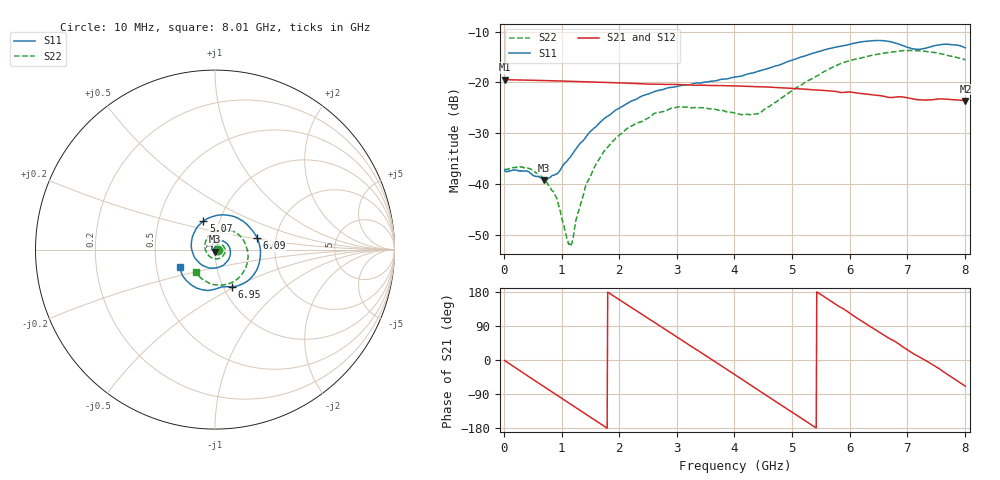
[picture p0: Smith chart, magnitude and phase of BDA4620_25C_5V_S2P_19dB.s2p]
!Agilent Technologies,E5071B,MY42404982,A.09.10
!Date: Wed May 06 09:02:22 2026
!Data & Calibration Information:
!Freq	S11:SOLT2(ON)	S21:SOLT2(ON)	S12:SOLT2(ON)	S22:SOLT2(ON)
# Hz S RI R 50
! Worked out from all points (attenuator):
!   801 points, 10 MHz to 8.01 GHz, reference 50 ohm
!   highest |S21| = -19.42 dB at 10 MHz (marker M1); lowest = -23.6 dB at 8.01 GHz (marker M2)
!   lowest |S11| = -39.2 dB at 700 MHz (marker M3), VSWR 1.02, Z = 49.8 - j1.08 ohm
!   |S11| at or under -10 dB: start of sweep to end of sweep
!   |S22| runs from -52.1 to -13.7 dB; largest |S21 - S12| = 0.00044
!   S11 on the Smith chart (normalised r, x): 10 MHz: 1.03, -0.00; 5.07 GHz: 0.84, +0.27; 6.09 GHz: 1.60, +0.22; 6.95 GHz: 1.10, -0.48; 8.01 GHz: 0.66, -0.14
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1e7  0.0137 -0.000932  0.1069 -0.00227  0.1071 -0.00226  0.014 -0.000475
4.1e8  0.00916 -0.00982  0.0785 -0.0703  0.0786 -0.0705  0.0135 -0.00511
7e8  -0.0015 -0.0108  0.0339 -0.0988  0.0339 -0.099  0.00854 -0.00729
9e8  -0.0103 -0.0072  -0.00221 -0.1037  -0.00227 -0.1039  0.00335 -0.0068
1.14e9  -0.0176 0.00455  -0.0438 -0.093  -0.044 -0.0932  -0.0021 -0.00153
1.19e9  -0.0183 0.00799  -0.0516 -0.0886  -0.0518 -0.0887  -0.00286 0.000131
1.35e9  -0.0184 0.0186  -0.0736 -0.0705  -0.0737 -0.0706  -0.00443 0.00544
1.56e9  -0.012 0.0334  -0.0931 -0.0393  -0.0932 -0.0393  -0.00381 0.0139
1.83e9  0.00664 0.0473  -0.0996 0.00681  -0.0997 0.00684  0.00279 0.024
2.15e9  0.0392 0.0492  -0.08 0.0575  -0.08 0.0576  0.0183 0.0307
2.68e9  0.0834 0.00493  -0.00398 0.096  -0.00396 0.0962  0.0466 0.0191
3.06e9  0.0779 -0.051  0.0547 0.0781  0.0549 0.0781  0.0571 -0.00766
4.01e9  -0.0762 -0.0835  0.0719 -0.0582  0.072 -0.0584  -0.0133 -0.0484
4.43e9  -0.1299 -0.000367  0.0146 -0.0895  0.0147 -0.0896  -0.0486 -0.0114
5.07e9  -0.0652 0.1576  -0.071 -0.0504  -0.0712 -0.0505  -0.0239 0.085
5.35e9  0.018 0.1919  -0.0841 -0.0112  -0.0842 -0.0113  0.0241 0.1064
6.09e9  0.2349 0.0645  -0.0329 0.0724  -0.0329 0.0724  0.1633 0.0436
6.39e9  0.2499 -0.0599  0.0063 0.0753  0.00616 0.0754  0.1836 -0.0236
6.68e9  0.1872 -0.1702  0.038 0.0605  0.0381 0.0607  0.173 -0.0948
6.95e9  0.0943 -0.207  0.0608 0.038  0.0608 0.038  0.1351 -0.1543
7.59e9  -0.0795 -0.2219  0.0616 -0.0311  0.0617 -0.0312  -0.0253 -0.1896
8.01e9  -0.1951 -0.0993  0.0233 -0.0616  0.0235 -0.0618  -0.1086 -0.1264
